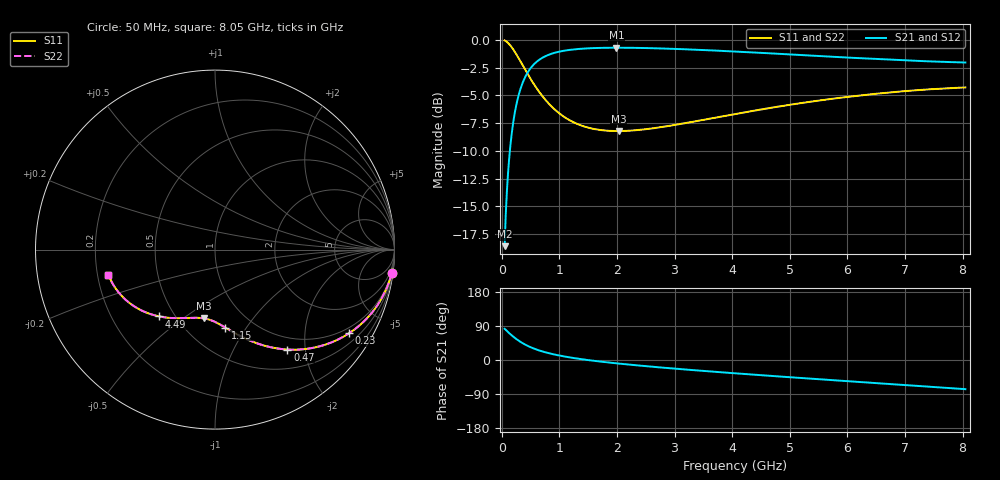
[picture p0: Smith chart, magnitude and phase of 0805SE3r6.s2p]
! AVX Thin Film Operation		Date: August 2001
! Description: Accu-P® Series, Thin Film, SMD, RF Capacitor
! Part Number: 08051J3R6ABT
! 50 MHz  -  8.05 GHz
! Serial Measurements
# mhz S db R 50
!	S11		S21		S12		S22
!	dB	Phase	dB	Phase	dB	Phase	dB	Phase
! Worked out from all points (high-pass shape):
!   401 points, 50 MHz to 8.05 GHz, reference 50 ohm
!   highest |S21| = -0.71 dB at 1.99 GHz (marker M1); lowest = -18.6 dB at 50 MHz (marker M2)
!   |S21| within 3 dB of the highest: 375.8 MHz to end of sweep
!   lowest |S11| = -8.2 dB at 2.03 GHz (marker M3), VSWR 2.27, Z = 33.3 - j30 ohm
!   |S11| at or under -10 dB: nowhere
!   |S22| runs from -8.2 to -0.1 dB; largest |S21 - S12| = 0
!   S11 on the Smith chart (normalised r, x): 50 MHz: 1, -15; 230 MHz: 0.80, -3.31; 470 MHz: 0.79, -1.67; 1.15 GHz: 0.75, -0.81; 4.49 GHz: 0.41, -0.40; 8.05 GHz: 0.25, -0.11
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50  -0.06 -7.6  -18.59 82.4  -18.59 82.4  -0.06 -7.6
70  -0.12 -10.5  -15.73 79.5  -15.73 79.5  -0.12 -10.5
110  -0.28 -16.3  -11.98 73.7  -11.98 73.7  -0.28 -16.3
150  -0.51 -21.9  -9.54 68.1  -9.54 68.1  -0.51 -21.9
190  -0.79 -27.1  -7.79 62.9  -7.79 62.9  -0.79 -27.1
230  -1.11 -32.0  -6.49 58.0  -6.49 58.0  -1.11 -32.0
330  -1.99 -42.6  -4.35 47.4  -4.35 47.4  -1.99 -42.6
470  -3.26 -54.1  -2.78 35.9  -2.78 35.9  -3.26 -54.1
610  -4.40 -62.7  -1.96 27.3  -1.96 27.3  -4.40 -62.7
750  -5.36 -69.3  -1.50 20.6  -1.50 20.6  -5.36 -69.3
930  -6.32 -76.0  -1.16 14.0  -1.16 14.0  -6.32 -76.0
1150  -7.16 -82.3  -0.93 7.6  -0.93 7.6  -7.16 -82.4
1390  -7.74 -87.9  -0.81 2.0  -0.81 2.0  -7.74 -87.9
1990  -8.22 -98.7  -0.71 -8.8  -0.71 -8.8  -8.22 -98.7
2030  -8.22 -99.4  -0.71 -9.4  -0.71 -9.4  -8.22 -99.4
2730  -7.89 -109.2  -0.78 -19.3  -0.78 -19.3  -7.89 -109.2
3370  -7.33 -117.2  -0.89 -27.3  -0.89 -27.3  -7.33 -117.2
4050  -6.69 -125.0  -1.06 -35.1  -1.06 -35.1  -6.69 -125.0
4490  -6.29 -129.8  -1.17 -39.9  -1.17 -39.9  -6.29 -129.8
5390  -5.56 -139.4  -1.43 -49.5  -1.43 -49.5  -5.56 -139.4
6730  -4.75 -153.2  -1.79 -63.3  -1.79 -63.3  -4.75 -153.2
8050  -4.29 -166.8  -2.05 -76.9  -2.05 -76.9  -4.29 -166.8
